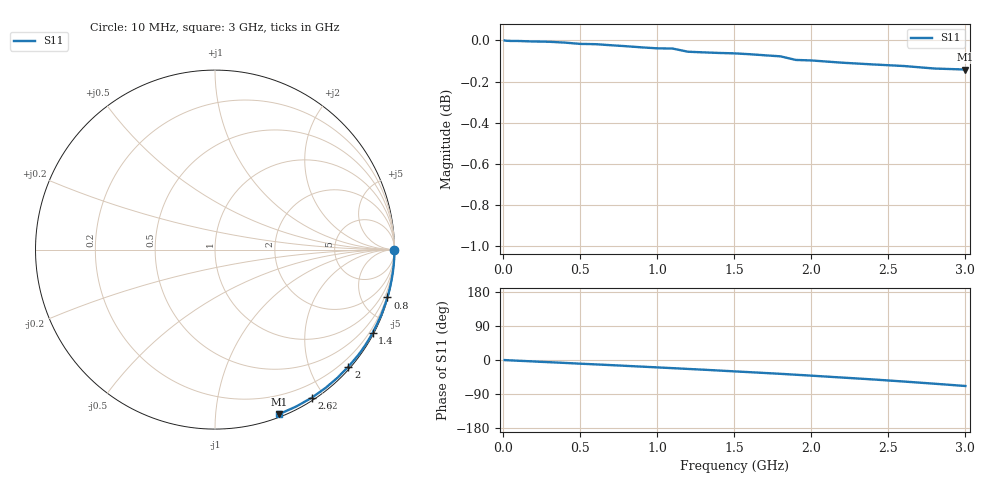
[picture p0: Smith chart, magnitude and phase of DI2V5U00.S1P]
! SIEMENS Small Signal Semiconductors
! BAV99
! Silicon Switching Diode in SOT23
! VR = 2.5 V
! S-Parameters:  May  1995
# GHz  S  MA  R  50
!  f  S11
! GHz  MAG  ANG
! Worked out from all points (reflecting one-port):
!   30 points, 10 MHz to 3 GHz, reference 50 ohm
!   lowest |S11| = -0.1 dB at 3 GHz (marker M1), VSWR 122.84, Z = 1.28 - j73.3 ohm
!   phase of S11 starts at -0 deg and turns -68 deg over the sweep
!   S11 on the Smith chart (normalised r, x): 10 MHz: open; 800 MHz: 0.09, -7.35; 1.4 GHz: 0.06, -4.04; 2 GHz: 0.04, -2.65; 2.6 GHz: 0.03, -1.85; 3 GHz: 0.03, -1.47
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0.01  1 -0.2
0.1  0.9997 -2.0
0.15  0.9995 -2.9
0.2  0.9994 -3.9
0.25  0.9993 -4.9
0.3  0.9993 -5.8
0.4  0.9988 -7.7
0.5  0.9981 -9.7
0.6  0.9979 -11.6
0.7  0.9973 -13.5
0.8  0.9968 -15.5
0.9  0.9961 -17.5
1  0.9956 -19.5
1.1  0.9955 -21.5
1.2  0.9937 -23.6
1.3  0.9933 -25.6
1.4  0.993 -27.8
1.5  0.9928 -30.0
1.6  0.9923 -32.1
1.7  0.9917 -34.3
1.8  0.9911 -36.5
1.9  0.9891 -38.9
2  0.9889 -41.3
2.2  0.9876 -46.3
2.4  0.9867 -51.3
2.6  0.9858 -56.8
2.8  0.9844 -62.6
3  0.9839 -68.6
